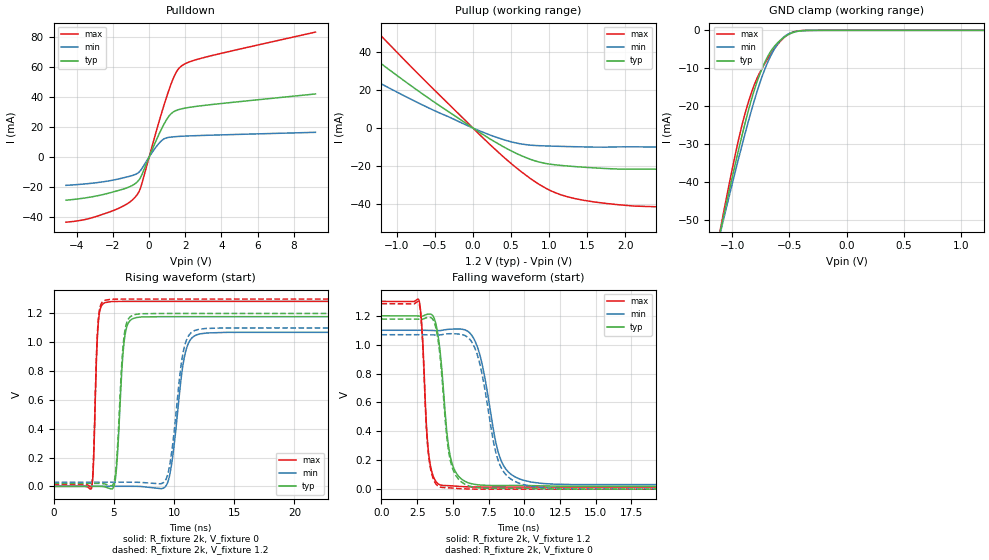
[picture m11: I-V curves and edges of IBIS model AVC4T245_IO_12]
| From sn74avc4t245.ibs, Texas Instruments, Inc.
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[Model]   AVC4T245_IO_12
Model_type  I/O
Vinl=0.385
Vinh=0.845
Enable   Active-Low
Vref =   0
Rref =   2000
Cref =   15p
Vmeas =   0.6
| variable   typ   min   max
C_comp   5.32pF   4.67pF   5.87pF
| C_pullup   5.80pF   3.90pF   7.86pF
| C_pulldown   5.35pF   4.78pF   7.04pF
| C_tri-state   5.32pF   4.67pF   5.87pF
[Temperature Range]   40   100   -40
| Ambient temperature   25   85   -40
[Voltage range]   1.2   1.1   1.3
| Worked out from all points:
|   slope of the pulldown table from 0 to 0.18 V, typ, clamps not added: 34.6 ohm
|   slope of the pullup table from 0 to 0.18 V, typ, clamps not added: 38.6 ohm
|   GND clamp passes 1 mA (typ) near -0.50 V on its own axis
|   rising waveform, R_fixture 2k, V_fixture 0: 20-80 % time 470ps typ, 867ps min, 282ps max; typ from 0 V to 1.18 V
|   falling waveform, R_fixture 2k, V_fixture 1.2: 20-80 % time 670ps typ, 1.21ns min, 400ps max; typ from 1.2 V to 0.02 V
|   rising waveform, R_fixture 2k, V_fixture 1.2: 20-80 % time 464ps typ, 850ps min, 280ps max; typ from 0.02 V to 1.2 V
|   falling waveform, R_fixture 2k, V_fixture 0: 20-80 % time 669ps typ, 1.21ns min, 398ps max; typ from 1.18 V to 0 V
[GND Clamp]
| AVC4T245_IO_12
|   Voltage   I(typ)   I(min)   I(max)
-4.6V     -600.6mA   -549.4mA   -665.2mA
-1.095V   -51.67mA   -52.21mA   -50.99mA
-1.07V    -48.21mA   -49.07mA   -47.1mA
-940mV    -30.91mA   -33.25mA   -28.18mA
-840mV    -19.08mA   -21.94mA   -17.15mA
-775mV    -12.89mA   -15.38mA   -12.1mA
-695mV    -7.221mA   -8.795mA   -7.744mA
-615mV    -3.667mA   -4.134mA   -4.191mA
-545mV    -1.809mA   -1.655mA   -1.862mA
-465mV    -549.4uA   -452.9uA   -430.6uA
-360mV    -50.53uA   -51.21uA   -21.62uA
1.2V      713.5pA    34.31nA    67.13pA
[Pulldown]
| AVC4T245_IO_12
|   Voltage   I(typ)   I(min)   I(max)
-4.6V     -28.79mA   -18.92mA   -43.46mA
-3.41V    -27.05mA   -17.8mA    -41.31mA
-2.035V   -23.45mA   -15.53mA   -35.96mA
-1.17V    -20.3mA    -13.14mA   -30.86mA
-680mV    -16.87mA   -11.13mA   -25.38mA
-435mV    -12.68mA   -8.327mA   -19.06mA
440mV     12.38mA    7.543mA    19.04mA
955mV     24.67mA    12.69mA    39.57mA
1.42V     30.53mA    13.49mA    54.64mA
1.79V     32.04mA    13.78mA    60.61mA
3.17V     34.51mA    14.41mA    66.63mA
9.2V      41.96mA    16.4mA     83.17mA
[Pullup]
| AVC4T245_IO_12
|   Voltage   I(typ)   I(min)   I(max)
-4.6V     40.24mA    7.956mA    186.3mA
-4.08V    45.4mA     8.808mA    167.8mA
-3.73V    53.63mA    9.647mA    154.2mA
-2.685V   79.31mA    16.98mA    111.4mA
-2.57V    75.87mA    21.96mA    106.5mA
-2.565V   75.72mA    49.43mA    106.3mA
-1.845V   53.66mA    37.03mA    75.82mA
-1.36V    38.76mA    26.71mA    55.3mA
575mV     -13.51mA   -7.977mA   -21.19mA
1.01V     -19.08mA   -9.527mA   -32.92mA
1.455V    -20.71mA   -9.971mA   -38.21mA
9.2V      -28.28mA   -12.48mA   -52.65mA
[Ramp]
| AVC4T245_IO_12
| variable   typ   min   max
dV/dt_r   0.72/4.83E-10   0.65/8.83E-10   0.78/2.91E-10
dV/dt_f   0.72/6.79E-10   0.65/1.23E-09   0.78/4.10E-10
R_load = 2k
[Rising Waveform]
| AVC4T245_IO_12
R_fixture =   2k
C_fixture =   0
L_fixture =   0
V_fixture =   0
V_fixture_min = 0
V_fixture_max = 0
|   Time   V(typ)   V(min)   V(max)
0s        18.11nV    102nV      416.8pV
3.155ns   606.6uV    -113.6uV   -13.8mV
3.7ns     440.2uV    151.1uV    1.116V
4.285ns   -4.158mV   163.3uV    1.275V
5.105ns   33.86mV    467.9uV    1.283V
5.86ns    1.003V     359.2uV    1.284V
6.635ns   1.166V     221.8uV    1.284V
9.455ns   1.178V     21.81mV    1.284V
11.89ns   1.178V     1.052V     1.284V
40ns      1.178V     1.069V     1.284V
[Falling Waveform]
| AVC4T245_IO_12
R_fixture =   2k
C_fixture =   0
L_fixture =   0
V_fixture =   1.2
V_fixture_min = 1.1
V_fixture_max = 1.3
|   Time   V(typ)   V(min)   V(max)
0s        1.2V       1.1V       1.3V
2.635ns   1.198V     1.1V       1.304V
3.305ns   1.212V     1.099V     245.8mV
4.12ns    941.2mV    1.098V     29.57mV
4.675ns   313.6mV    1.106V     24.26mV
5.235ns   111.6mV    1.109V     20.63mV
6.58ns    32.59mV    1.019V     15.06mV
8.28ns    24.97mV    223.1mV    14.53mV
9.92ns    25.71mV    62.21mV    14.51mV
40ns      20.14mV    28.75mV    14.5mV
[Rising Waveform]
| AVC4T245_IO_12
R_fixture =   2k
C_fixture =   0
L_fixture =   0
V_fixture =   1.2
V_fixture_min = 1.1
V_fixture_max = 1.3
|   Time   V(typ)   V(min)   V(max)
0s        20.14mV    28.74mV    14.5mV
3.155ns   20.71mV    28.68mV    2.256mV
3.695ns   20.45mV    28.94mV    1.135V
4.275ns   16.13mV    28.92mV    1.292V
5.08ns    51.82mV    29.12mV    1.299V
5.83ns    1.023V     28.88mV    1.3V
6.605ns   1.188V     28.65mV    1.3V
9.375ns   1.2V       55.8mV     1.3V
11.74ns   1.2V       1.083V     1.3V
40ns      1.2V       1.1V       1.3V
[Falling Waveform]
| AVC4T245_IO_12
R_fixture =   2k
C_fixture =   0
L_fixture =   0
V_fixture =   0
V_fixture_min = 0
V_fixture_max = 0
|   Time   V(typ)   V(min)   V(max)
0s        1.178V     1.069V     1.284V
2.635ns   1.177V     1.069V     1.287V
3.3ns     1.189V     1.068V     230.9mV
4.1ns     923.3mV    1.068V     15.16mV
4.65ns    298mV      1.076V     9.669mV
5.22ns    92.51mV    1.075V     5.59mV
6.675ns   11.25mV    941.4mV    382.8uV
8.305ns   4.999mV    164.9mV    26.47uV
9.865ns   5.435mV    33.57mV    6.981uV
40ns      79.55nV    4.482uV    24.51nV
